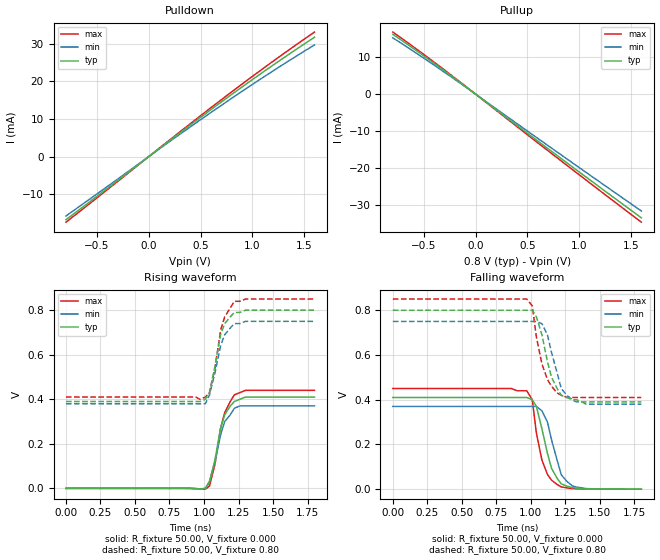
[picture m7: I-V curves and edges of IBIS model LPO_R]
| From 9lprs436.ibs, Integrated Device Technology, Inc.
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|   Model LPO_R
[Model]   LPO_R
Model_type   Output
Polarity   Inverting
Vmeas =   0.40V
Cref =   2.00pF
Rref =  0.000
Vref =   0.40V
C_comp   3.40pF   2.85pF   3.95pF
[Temperature Range]   27.00   70.00   0.000
[Voltage Range]   0.80V   0.75V   0.85V
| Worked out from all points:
|   slope of the pulldown table from 0 to 0.12 V, typ, clamps not added: 47.2 ohm
|   slope of the pullup table from 0 to 0.12 V, typ, clamps not added: 47 ohm
|   rising waveform, R_fixture 50.00, V_fixture 0.000: 20-80 % time 87.8ps typ, 89ps min, 88.5ps max; typ from 0 V to 0.41 V
|   rising waveform, R_fixture 50.00, V_fixture 0.80: 20-80 % time 82.8ps typ, 88ps min, 81.3ps max; typ from 0.39 V to 0.8 V
|   falling waveform, R_fixture 50.00, V_fixture 0.000: 20-80 % time 103ps typ, 94.1ps min, 86.9ps max; typ from 0.41 V to 0 V
|   falling waveform, R_fixture 50.00, V_fixture 0.80: 20-80 % time 106ps typ, 93ps min, 93ps max; typ from 0.8 V to 0.39 V
[Pulldown]
| voltage   I(typ)   I(min)   I(max)
-800mV    -16.76mA   -15.78mA   -17.43mA
600mV     12.47mA    11.71mA    12.99mA
1.1V      22.38mA    20.97mA    23.32mA
1.6V      31.7mA     29.66mA    33.08mA
[Pullup]
| voltage   I(typ)   I(min)   I(max)
-800mV    16.2mA     15.25mA    16.8mA
-300mV    6.28mA     5.91mA     6.52mA
700mV     -14.78mA   -13.94mA   -15.33mA
1.6V      -33.46mA   -31.61mA   -34.64mA
[Ramp]
| variable   typ   min   max
dV/dt_r   0.25/88.04p   0.22/90.43p   0.27/84.29p
dV/dt_f   0.25/89.71p   0.22/94.68p   0.27/86.85p
R_load = 50.00
[Rising Waveform]
R_fixture = 50.00
V_fixture = 0.000
V_fixture_min = 0.000
V_fixture_max = 0.000
| time   V(typ)   V(min)   V(max)
0s        0V         0V         0V
1.01ns    -1.57mV    620uV      -3.6mV
1.04ns    28.04mV    32.36mV    11.03mV
1.08ns    130mV      120mV      110mV
1.12ns    270mV      240mV      270mV
1.15ns    330mV      300mV      340mV
1.19ns    370mV      330mV      390mV
1.22ns    390mV      360mV      420mV
1.3ns     410mV      370mV      440mV
1.8ns     410mV      370mV      440mV
[Rising Waveform]
R_fixture = 50.00
V_fixture = 0.80
V_fixture_min = 0.75
V_fixture_max = 0.85
| time   V(typ)   V(min)   V(max)
0s        390mV      380mV      410mV
940ps     390mV      380mV      410mV
970ps     390mV      380mV      400mV
1.01ns    400mV      380mV      410mV
1.04ns    430mV      420mV      430mV
1.08ns    550mV      520mV      540mV
1.12ns    690mV      640mV      710mV
1.15ns    740mV      690mV      770mV
1.22ns    790mV      740mV      840mV
1.8ns     800mV      750mV      850mV
[Falling Waveform]
R_fixture = 50.00
V_fixture = 0.000
V_fixture_min = 0.000
V_fixture_max = 0.000
| time   V(typ)   V(min)   V(max)
0s        410mV      370mV      450mV
970ps     410mV      370mV      440mV
1.01ns    400mV      370mV      400mV
1.04ns    370mV      370mV      250mV
1.08ns    270mV      350mV      130mV
1.12ns    160mV      300mV      65.86mV
1.15ns    92.88mV    220mV      40.16mV
1.22ns    23.85mV    64.57mV    9.99mV
1.3ns     7.09mV     14.76mV    2.7mV
1.8ns     72.44uV    110uV      52.48uV
[Falling Waveform]
R_fixture = 50.00
V_fixture = 0.80
V_fixture_min = 0.75
V_fixture_max = 0.85
| time   V(typ)   V(min)   V(max)
0s        800mV      750mV      850mV
970ps     800mV      750mV      850mV
1.01ns    800mV      750mV      820mV
1.04ns    770mV      750mV      680mV
1.08ns    690mV      740mV      560mV
1.15ns    500mV      610mV      460mV
1.19ns    450mV      520mV      430mV
1.22ns    420mV      450mV      420mV
1.33ns    400mV      390mV      410mV
1.8ns     390mV      380mV      410mV
